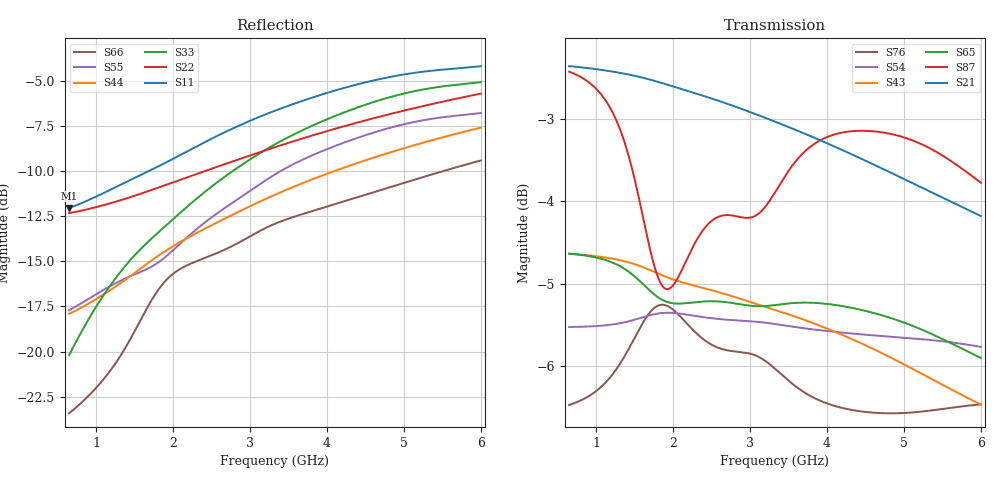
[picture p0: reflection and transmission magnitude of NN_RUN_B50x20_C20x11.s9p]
! IGNION VIRTUAL ANTENNA LIBRARY
! NN_RUN_B50x20_C20x11
! Virtual Antenna™ RUN mXTEND™: NN02-224 12.0 mm x 3.0 mm x 2.4 mm
! https://ignion.io/product/run-mxtend/
! Board: 50 mm x 20 mm
! Clearance Area: 20 mm x 11 mm
! Feeding line: L-shape; 11mm x 2mm and 5mm x 2mm
! Applications: Fleet management, IoT
! Frequency range 0.65GHz to 6GHz, step 10MHz
! Number of ports 9
! This product and its use is protected by at least one or more of the following patents and patent
! applications US 8,203,492 B2; US 8,237,615 B2; PCT/EP2013/064692; WO 2014/012842 A1; US 2019/190122 A1;
! US 62/072,671; and other domestic and international patents pending. Additional information about
! patents related to this product is available at https://ignion.io/files/Patent-list-NN.pdf, all
! rights reserved. Copyright, Ignion 2021.
! Need more help? Your platform is much different than these examples in the manual? Use our
! Fast Track service (https://ignion.io/fast-track/), for free, and get a personalized antenna design in
! just 24 hours.
! Touchstone port 1 = "Series Port"
! Touchstone port 2 = "Shunt Port"
! Touchstone port 3 = "Series Port"
! Touchstone port 4 = "Shunt Port"
! Touchstone port 5 = "Series Port"
! Touchstone port 6 = "Shunt Port"
! Touchstone port 7 = "Series Port"
! Touchstone port 8 = "Shunt Port"
! Touchstone port 9 = "Series Port"
! IE3D S-Parameters Output Version 2.0
# GHZ S MA R 50
! Nport = 9
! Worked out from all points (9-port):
!   536 points, 650 MHz to 6 GHz, reference 50 ohm
!   strongest paths, dB at 650 MHz, 1.99 GHz, 3.33 GHz, 4.67 GHz, 6 GHz:
!     S21: -2.4, -2.6, -3.0, -3.6, -4.2
!     S87: -2.4, -5.0, -3.9, -3.2, -3.8
!     S65: -4.6, -5.2, -5.3, -5.4, -5.9
!     S43: -4.6, -4.9, -5.3, -5.8, -6.5
!     S54: -5.5, -5.4, -5.5, -5.6, -5.8
!     S76: -6.5, -5.3, -6.0, -6.6, -6.5
!   lowest |S11| = -12.0 dB at 650 MHz (marker M1), VSWR 1.67, Z = 31.1 + j7.7 ohm
!   |S11| at or under -10 dB: start of sweep to 1.683 GHz
